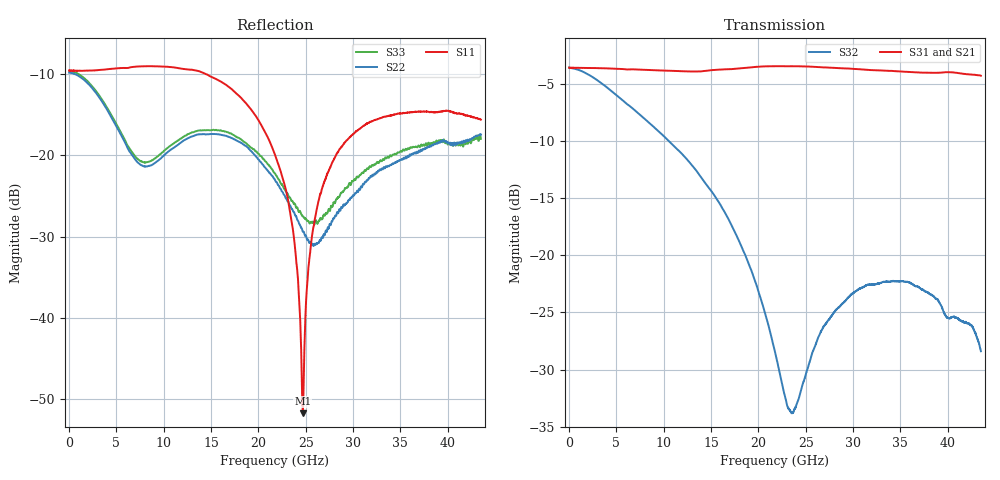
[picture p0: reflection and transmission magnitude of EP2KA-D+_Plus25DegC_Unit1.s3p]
!Keysight Technologies,N5244A,MY52442000,A.10.40.14
!Date: Thursday, March 23, 2017 16:07:54
!DIE PROBE
!Correction: S11(Full 3 Port(1,2,3))
!S12(Full 3 Port(1,2,3))
!S13(Full 3 Port(1,2,3))
!S21(Full 3 Port(1,2,3))
!S22(Full 3 Port(1,2,3))
!S23(Full 3 Port(1,2,3))
!S31(Full 3 Port(1,2,3))
!S32(Full 3 Port(1,2,3))
!S33(Full 3 Port(1,2,3))
!S3P File: Measurements: <S11,S12,S13>,
!<S21,S22,S23>,
!<S31,S32,S33>:
# Hz S  dB  R 50
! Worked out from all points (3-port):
!   4350 points, 10 MHz to 43.5 GHz, reference 50 ohm
!   strongest paths, dB at 10 MHz, 10.88 GHz, 21.76 GHz, 32.63 GHz, 43.5 GHz:
!     S31: -3.6, -3.9, -3.4, -3.8, -4.3
!     S21: -3.6, -3.9, -3.5, -3.8, -4.3
!     S32: -3.6, -10.3, -28.5, -22.5, -28.4
!   lowest |S11| = -51.7 dB at 24.69 GHz (marker M1), VSWR 1.01, Z = 49.9 + j0.248 ohm
!   |S11| at or under -10 dB: 14.39 GHz to end of sweep
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1e7  -9.61 -179.9  -3.49 0.0  -3.57 -0.1
     -3.56 -0.1  -9.86 179.8  -3.64 -0.3
     -3.58 -0.2  -3.56 -0.1  -9.64 180.0
4.16e9  -9.43 167.0  -3.62 -38.8  -3.64 -38.4
        -3.62 -38.7  -14.69 128.4  -5.41 -58.8
        -3.64 -38.5  -5.40 -58.9  -14.45 129.4
1.036e10  -9.14 137.3  -3.85 -94.9  -3.84 -94.6
          -3.85 -94.9  -19.69 157.1  -9.85 -127.4
          -3.84 -94.6  -9.85 -127.4  -19.14 157.9
2.176e10  -19.96 46.0  -3.45 160.4  -3.45 160.6
          -3.45 160.4  -23.03 85.1  -28.47 81.4
          -3.44 160.6  -28.48 81.4  -22.25 91.8
2.369e10  -29.48 31.3  -3.45 141.4  -3.45 141.8
          -3.45 141.4  -26.95 82.3  -33.71 0.1
          -3.45 141.8  -33.71 -0.0  -25.89 94.4
2.469e10  -51.72 106.8  -3.47 131.6  -3.46 132.0
          -3.47 131.6  -29.39 87.5  -31.26 -43.0
          -3.46 132.0  -31.25 -42.9  -27.50 100.8
2.581e10  -28.83 -178.4  -3.50 120.6  -3.50 121.0
          -3.51 120.6  -31.16 107.3  -28.29 -71.5
          -3.50 121.0  -28.30 -71.6  -28.25 116.3
2.853e10  -19.35 159.0  -3.63 94.2  -3.61 94.7
          -3.63 94.2  -26.71 130.1  -24.52 -113.1
          -3.61 94.7  -24.52 -113.1  -25.13 135.3
3.663e10  -14.68 85.2  -4.00 16.1  -3.98 16.6
          -4.00 16.1  -19.80 71.3  -22.71 165.6
          -3.98 16.6  -22.70 165.6  -18.94 79.7
4.35e10  -15.64 23.3  -4.31 -53.0  -4.28 -52.9
         -4.31 -53.0  -17.46 16.4  -28.39 97.6
         -4.28 -52.9  -28.40 97.5  -18.00 28.0
